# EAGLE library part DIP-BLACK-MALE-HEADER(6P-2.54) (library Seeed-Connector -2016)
320020078
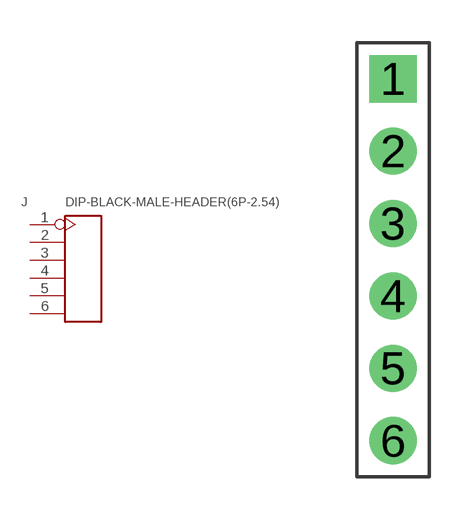
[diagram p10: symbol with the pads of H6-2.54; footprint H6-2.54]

Designator prefix J

## DIP-BLACK-MALE-HEADER(6P-2.54) (MPN: P125-1106A1BS116A1; VALUE: 6p-2.54)  [H6-2.54]
1  1
2  2
3  3
4  4
5  5
6  6

## Footprint H6-2.54 (pad centres in mm)
drill 0.889 pad 1.651 square: 1 0,6.35
drill 0.889 pad 1.651: 2 0,3.81; 3 0,1.27; 4 0,-1.27; 5 0,-3.81; 6 0,-6.35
